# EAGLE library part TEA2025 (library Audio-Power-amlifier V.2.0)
DUAL OR BRIDGE CONNECTION MODES FEW EXTERNAL COMPONENTS SUPPLY VOLTAGE DOWN TO 3V HIGH CHANNEL SEPARATION VERY LOW SWITCH ON/OFF NOISE MAX GAIN OF 45dB WITH ADJUST EXTERNAL RESISTOR SOFT CLIPPING THERMAL PROTECTION 3V < VCC < 15V P = 2 · 1W, VCC = 6V, RL = 4W P = 2 · 2.3W, VCC = 9V, RL = 4W P = 2 · 0.1W, VCC = 3V, RL = 4W
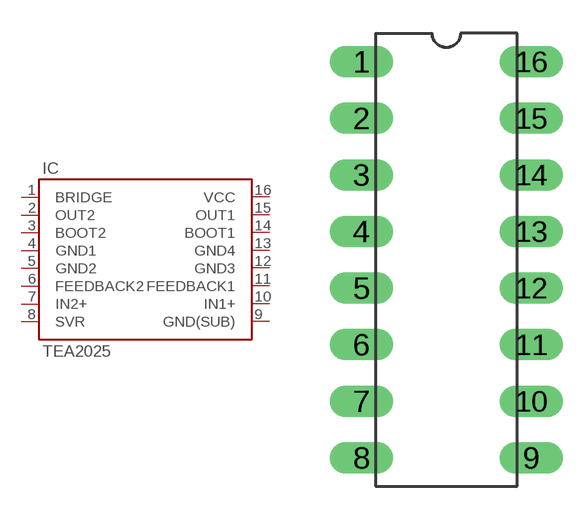
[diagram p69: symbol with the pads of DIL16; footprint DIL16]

Designator prefix IC

## TEA2025  [DIL16]
1  BRIDGE
2  OUT2
3  BOOT2
4  GND1
5  GND2
6  FEEDBACK2
7  IN2+
8  SVR
9  GND(SUB)
10  IN1+
11  FEEDBACK1
12  GND3
13  GND4
14  BOOT1
15  OUT1
16  VCC

## Footprint DIL16 (pad centres in mm)
drill 0.8 pad 1.422 long: 1 -3.81,8.89; 2 -3.81,6.35; 3 -3.81,3.81; 4 -3.81,1.27; 5 -3.81,-1.27; 6 -3.81,-3.81; 7 -3.81,-6.35; 8 -3.81,-8.89; 9 3.81,-8.89; 10 3.81,-6.35; 11 3.81,-3.81; 12 3.81,-1.27; 13 3.81,1.27; 14 3.81,3.81; 15 3.81,6.35; 16 3.81,8.89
